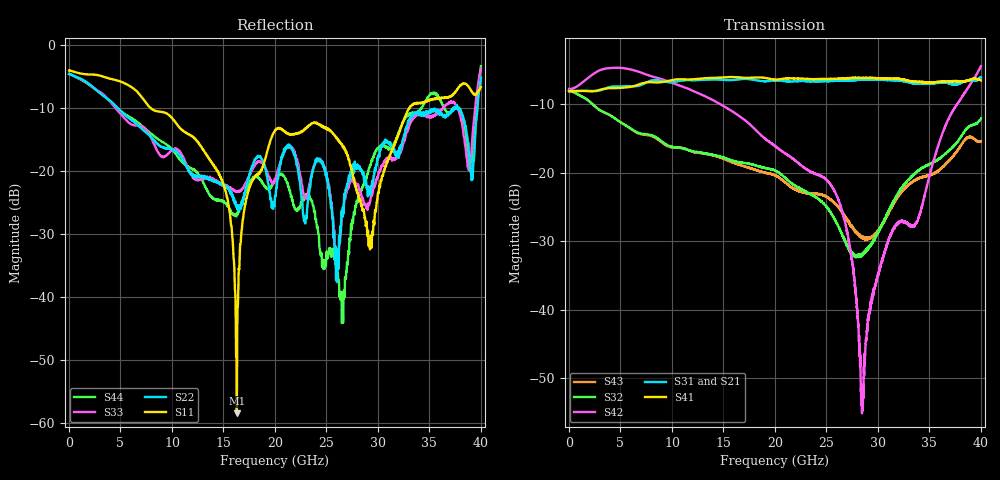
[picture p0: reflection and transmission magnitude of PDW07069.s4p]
!The following data was pulled from an Agilent PNA
!This sNp file was generated from the data in the RF Test software
!NOTE:  Smoothing/Math/Corrections applied on any given trace ARE included in the data saved here
# MHz S dB R 50
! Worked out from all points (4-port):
!   4000 points, 10 MHz to 40 GHz, reference 50 ohm
!   strongest paths, dB at 10 MHz, 10.01 GHz, 20.01 GHz, 30.01 GHz, 40 GHz:
!     S41: -8.1, -6.4, -6.4, -6.2, -6.5
!     S31: -8.0, -6.7, -6.5, -6.4, -6.0
!     S21: -8.0, -6.5, -6.7, -6.5, -6.4
!     S42: -7.7, -6.8, -16.1, -34.9, -4.4
!     S32: -8.0, -16.2, -19.7, -28.7, -12.0
!     S43: -8.0, -16.3, -20.4, -28.6, -15.4
!   lowest |S11| = -58.4 dB at 16.3 GHz (marker M1), VSWR 1.00, Z = 49.9 + j0.0995 ohm
!   |S11| at or under -10 dB: 7.966 GHz to 33.05 GHz (25.08 GHz wide, 122 % of centre)
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10  -3.96 -179.8  -8.03 -0.0  -8.01 0.1  -8.04 0.1
    -8.01 -0.1  -4.51 -179.7  -8.00 0.1  -7.78 0.5
    -8.01 -0.1  -7.98 0.2  -4.53 -179.6  -8.05 0.2
    -8.08 0.2  -7.75 0.6  -8.02 0.2  -4.52 -179.7
12850  -16.11 -59.8  -6.34 152.4  -6.41 153.1  -6.22 147.9
       -6.35 152.5  -20.88 -47.2  -17.06 66.5  -8.56 -155.3
       -6.41 153.2  -17.06 66.6  -21.31 -48.1  -17.13 65.9
       -6.22 148.1  -8.56 -155.2  -17.13 65.9  -21.17 -35.9
16300  -58.39 124.2  -6.36 91.3  -6.37 93.3  -6.01 85.6
       -6.37 91.4  -25.65 -39.6  -18.39 -5.7  -11.44 162.4
       -6.38 93.4  -18.39 -5.5  -23.17 -44.7  -18.70 -7.0
       -6.02 85.8  -11.44 162.5  -18.69 -7.0  -26.72 -63.6
20150  -13.25 -24.5  -6.71 23.6  -6.50 24.8  -6.36 17.3
       -6.73 23.7  -22.64 -98.3  -19.81 -96.6  -16.25 127.5
       -6.51 24.9  -19.79 -96.5  -20.77 -84.6  -20.49 -104.6
       -6.37 17.6  -16.25 127.6  -20.47 -104.4  -21.02 -80.4
26460  -15.73 -63.4  -6.59 -90.1  -6.53 -89.2  -6.21 -98.7
       -6.58 -89.8  -26.56 151.5  -28.86 58.0  -25.29 55.9
       -6.51 -89.0  -28.85 57.9  -27.98 -176.8  -25.64 46.2
       -6.19 -98.3  -25.27 56.4  -25.63 46.5  -39.98 154.1
28490  -26.12 -50.2  -6.48 -128.6  -6.39 -127.8  -6.13 -138.4
       -6.46 -128.4  -20.17 179.5  -31.98 -59.5  -55.67 -87.6
       -6.38 -127.5  -31.98 -59.4  -24.27 -168.0  -29.49 -43.2
       -6.14 -138.0  -54.52 -84.4  -29.58 -43.4  -22.58 106.4
40000  -6.59 -51.3  -6.38 -0.3  -6.00 -1.1  -6.46 -14.4
       -6.41 -0.0  -5.09 -50.9  -12.08 -76.0  -4.46 139.2
       -6.04 -0.8  -12.04 -75.9  -3.69 -44.7  -15.41 -76.2
       -6.47 -14.0  -4.41 139.1  -15.40 -76.6  -3.28 -62.9
